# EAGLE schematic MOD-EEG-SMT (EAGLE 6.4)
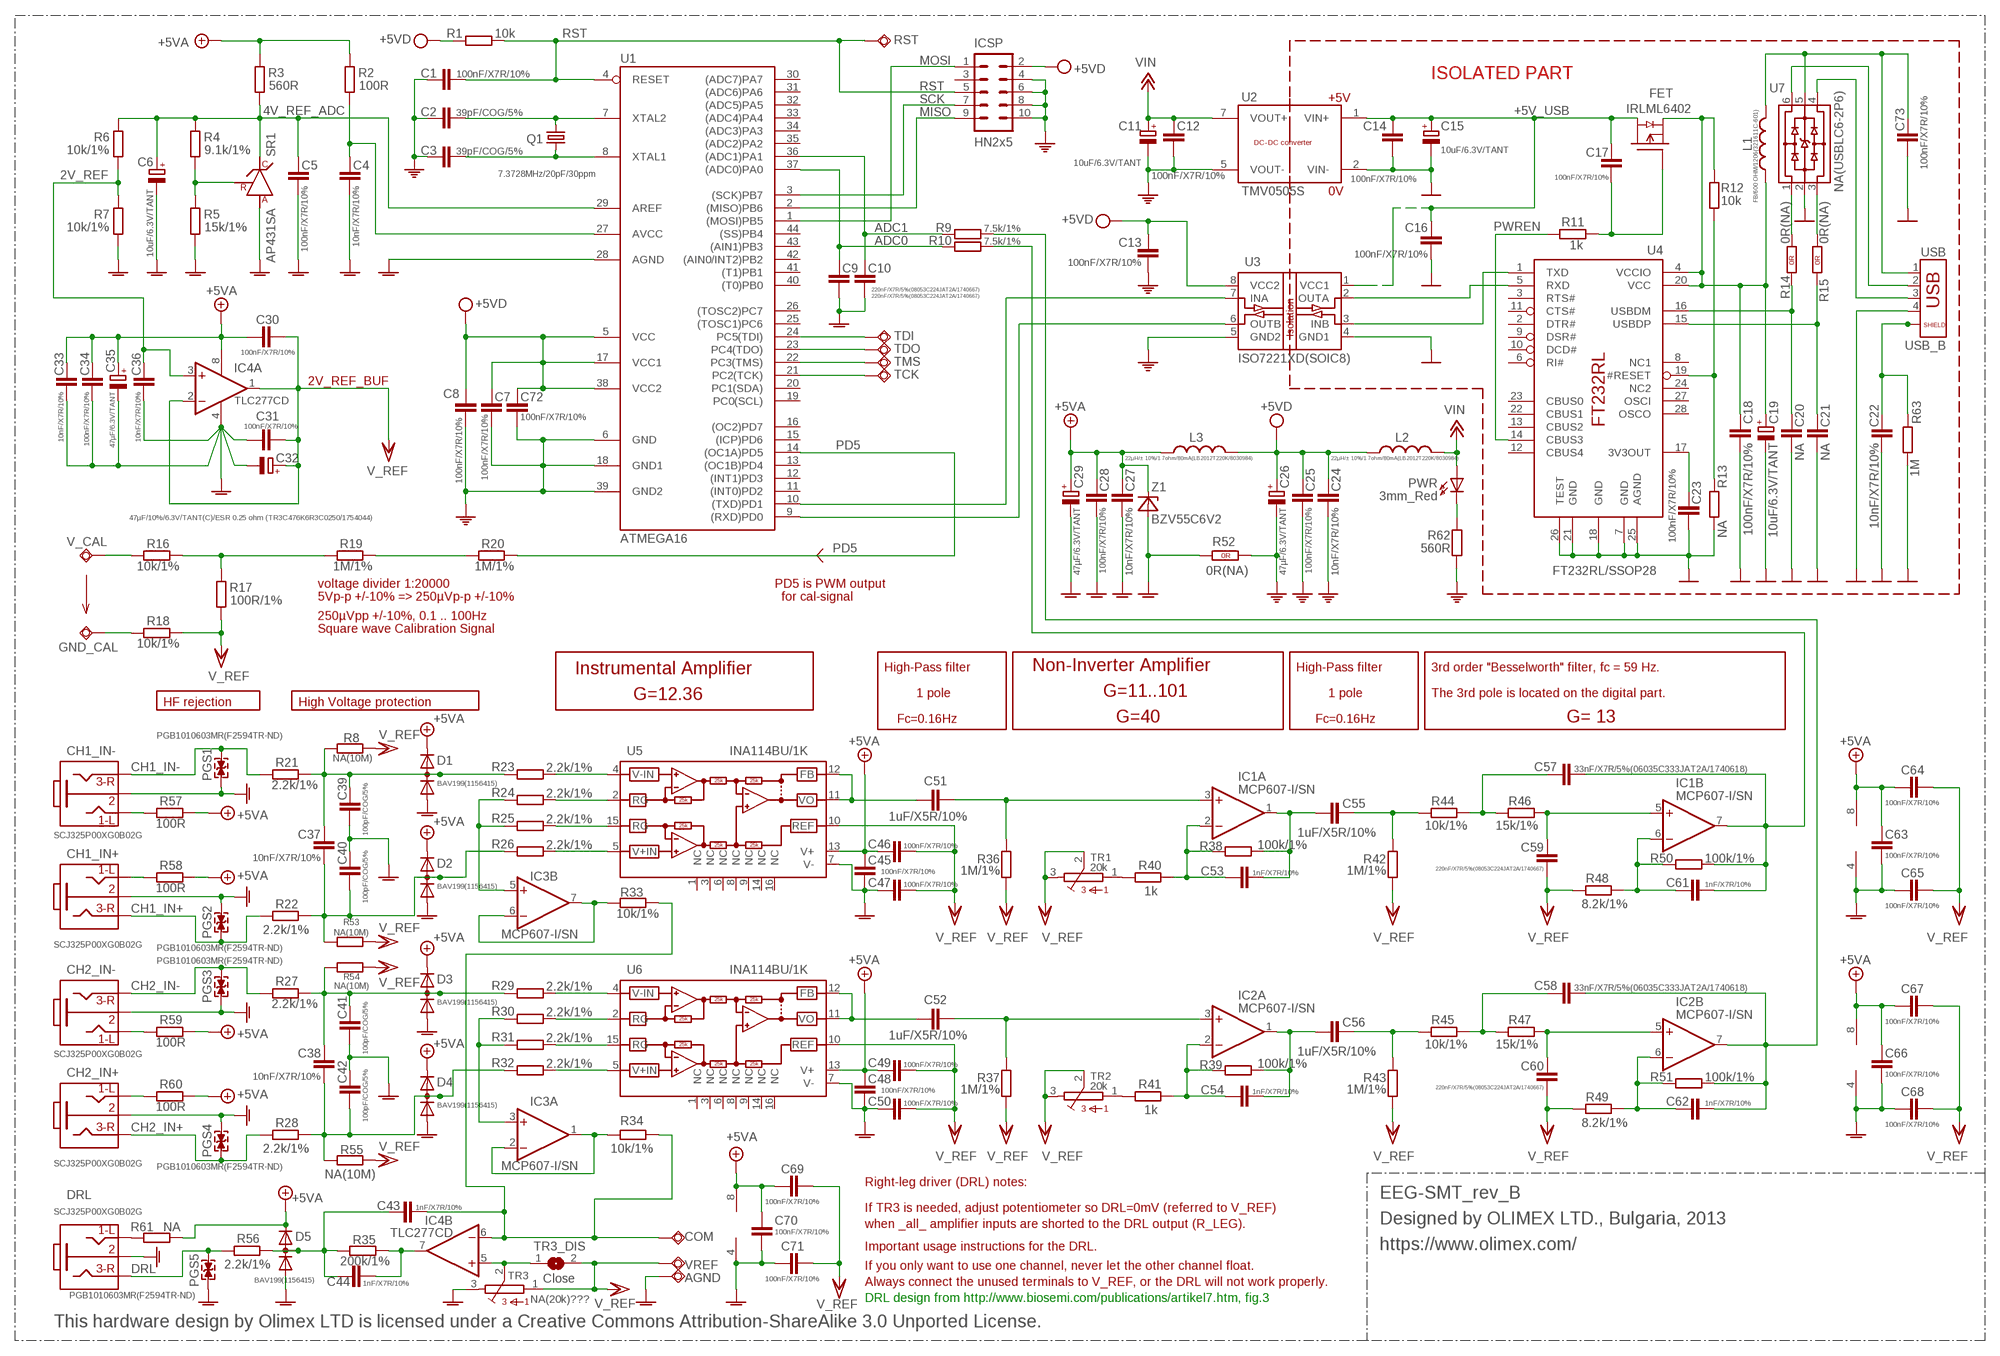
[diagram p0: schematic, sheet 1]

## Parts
AGND  TESTPAD3  [TEST_PAD40/70/SQUARE]
C1  100nF/X7R/10%  C-EUC0603_DWS  [C0603_DWS]
C2  39pF/COG/5%  C-EUC0603_DWS  [C0603_DWS]
C3  39pF/COG/5%  C-EUC0603_DWS  [C0603_DWS]
C4  10nF/X7R/10%  C-EUC0603_DWS  [C0603_DWS]
C5  100nF/X7R/10%  C-EUC0603_DWS  [C0603_DWS]
C6  10uF/6.3V/TANT  CPOL-EUCT3216  [CT3216]
C7  100nF/X7R/10%  C-EUC0603_DWS  [C0603_DWS]
C8  100nF/X7R/10%  C-EUC0603_DWS  [C0603_DWS]
C9  220nF/X7R/5%(08053C224JAT2A/1740667)  C-EUC0805_5MIL_DWS  [C0805_5MIL_DWS]
C10  220nF/X7R/5%(08053C224JAT2A/1740667)  C-EUC0805_5MIL_DWS  [C0805_5MIL_DWS]
C11  10uF/6.3V/TANT  CPOL-EUCT3216  [CT3216]
C12  100nF/X7R/10%  C-EUC0603_DWS  [C0603_DWS]
C13  100nF/X7R/10%  C-EUC0603_DWS  [C0603_DWS]
C14  100nF/X7R/10%  C-EUC0603_DWS  [C0603_DWS]
C15  10uF/6.3V/TANT  CPOL-EUCT3216  [CT3216]
C16  100nF/X7R/10%  C-EUC0603_DWS  [C0603_DWS]
C17  100nF/X7R/10%  C-EUC0603_DWS  [C0603_DWS]
C18  100nF/X7R/10%  C-EUC0603_DWS  [C0603_DWS]
C19  10uF/6.3V/TANT  CPOL-EUCT3216  [CT3216]
C20  NA  C-EUC0603_DWS_NA  [C0603_DWS_NA]
C21  NA  C-EUC0603_DWS_NA  [C0603_DWS_NA]
C22  10nF/X7R/10%  C-EUC0603_DWS  [C0603_DWS]
C23  100nF/X7R/10%  C-EUC0603_DWS  [C0603_DWS]
C24  10nF/X7R/10%  C-EUC0603_DWS  [C0603_DWS]
C25  100nF/X7R/10%  C-EUC0603_DWS  [C0603_DWS]
C26  47µF/6.3V/TANT  CPOL-EUCT3528  [CT3528]
C27  10nF/X7R/10%  C-EUC0603_DWS  [C0603_DWS]
C28  100nF/X7R/10%  C-EUC0603_DWS  [C0603_DWS]
C29  47µF/6.3V/TANT  CPOL-EUCT3528  [CT3528]
C30  100nF/X7R/10%  C-EUC0603_DWS  [C0603_DWS]
C31  100nF/X7R/10%  C-EUC0603_DWS  [C0603_DWS]
C32  47µF/10%/6.3V/TANT(C)/ESR 0.25 ohm (TR3C476K6R3C0250/1754044)  CPOL-EUCT6032  [CT6032]
C33  10nF/X7R/10%  C-EUC0603_DWS  [C0603_DWS]
C34  100nF/X7R/10%  C-EUC0603_DWS  [C0603_DWS]
C35  47µF/6.3V/TANT  CPOL-EUCT3528  [CT3528]
C36  10nF/X7R/10%  C-EUC0603_DWS  [C0603_DWS]
C37  10nF/X7R/10%  C-EUC0603_DWS  [C0603_DWS]
C38  10nF/X7R/10%  C-EUC0603_DWS  [C0603_DWS]
C39  100pF/COG/5%  C-EUC0603_DWS  [C0603_DWS]
C40  100pF/COG/5%  C-EUC0603_DWS  [C0603_DWS]
C41  100pF/COG/5%  C-EUC0603_DWS  [C0603_DWS]
C42  100pF/COG/5%  C-EUC0603_DWS  [C0603_DWS]
C43  1nF/X7R/10%  C-EUC0603_DWS  [C0603_DWS]
C44  1nF/X7R/10%  C-EUC0603_DWS  [C0603_DWS]
C45  100nF/X7R/10%  C-EUC0603_DWS  [C0603_DWS]
C46  100nF/X7R/10%  C-EUC0603_DWS  [C0603_DWS]
C47  100nF/X7R/10%  C-EUC0603_DWS  [C0603_DWS]
C48  100nF/X7R/10%  C-EUC0603_DWS  [C0603_DWS]
C49  100nF/X7R/10%  C-EUC0603_DWS  [C0603_DWS]
C50  100nF/X7R/10%  C-EUC0603_DWS  [C0603_DWS]
C51  1uF/X5R/10%  C-EUC0603_DWS  [C0603_DWS]
C52  1uF/X5R/10%  C-EUC0603_DWS  [C0603_DWS]
C53  1nF/X7R/10%  C-EUC0603_DWS  [C0603_DWS]
C54  1nF/X7R/10%  C-EUC0603_DWS  [C0603_DWS]
C55  1uF/X5R/10%  C-EUC0603_DWS  [C0603_DWS]
C56  1uF/X5R/10%  C-EUC0603_DWS  [C0603_DWS]
C57  33nF/X7R/5%(06035C333JAT2A/1740618)  C-EUC0603_DWS  [C0603_DWS]
C58  33nF/X7R/5%(06035C333JAT2A/1740618)  C-EUC0603_DWS  [C0603_DWS]
C59  220nF/X7R/5%(08053C224JAT2A/1740667)  C-EUC0805_5MIL_DWS  [C0805_5MIL_DWS]
C60  220nF/X7R/5%(08053C224JAT2A/1740667)  C-EUC0805_5MIL_DWS  [C0805_5MIL_DWS]
C61  1nF/X7R/10%  C-EUC0603_DWS  [C0603_DWS]
C62  1nF/X7R/10%  C-EUC0603_DWS  [C0603_DWS]
C63  100nF/X7R/10%  C-EUC0603_DWS  [C0603_DWS]
C64  100nF/X7R/10%  C-EUC0603_DWS  [C0603_DWS]
C65  100nF/X7R/10%  C-EUC0603_DWS  [C0603_DWS]
C66  100nF/X7R/10%  C-EUC0603_DWS  [C0603_DWS]
C67  100nF/X7R/10%  C-EUC0603_DWS  [C0603_DWS]
C68  100nF/X7R/10%  C-EUC0603_DWS  [C0603_DWS]
C69  100nF/X7R/10%  C-EUC0603_DWS  [C0603_DWS]
C70  100nF/X7R/10%  C-EUC0603_DWS  [C0603_DWS]
C71  100nF/X7R/10%  C-EUC0603_DWS  [C0603_DWS]
C72  100nF/X7R/10%  C-EUC0603_DWS  [C0603_DWS]
C73  100nF/X7R/10%  C-EUC0603_DWS  [C0603_DWS]
CH1_IN+  SCJ325P00XG0B02G  JACK-3PINPHONE_JACK-SMD  [PHONE_JACK-SMD]
CH1_IN-  SCJ325P00XG0B02G  JACK-3PINPHONE_JACK-SMD  [PHONE_JACK-SMD]
CH2_IN+  SCJ325P00XG0B02G  JACK-3PINPHONE_JACK-SMD  [PHONE_JACK-SMD]
CH2_IN-  SCJ325P00XG0B02G  JACK-3PINPHONE_JACK-SMD  [PHONE_JACK-SMD]
COM  TESTPAD3  [TEST_PAD40/70/SQUARE]
D1  BAV199(1156415)  DIODE_AC-AC_  [SOT23C(BAT54S)]
D2  BAV199(1156415)  DIODE_AC-AC_  [SOT23C(BAT54S)]
D3  BAV199(1156415)  DIODE_AC-AC_  [SOT23C(BAT54S)]
D4  BAV199(1156415)  DIODE_AC-AC_  [SOT23C(BAT54S)]
D5  BAV199(1156415)  DIODE_AC-AC_  [SOT23C(BAT54S)]
DRL  SCJ325P00XG0B02G  JACK-3PINPHONE_JACK-SMD  [PHONE_JACK-SMD]
FET  IRLML6402  [SOT23]
GND_CAL  TESTPAD3  [TEST_PAD40/70/SQUARE]
IC1  MCP607-I/SN  LM358D  [SO08]
IC2  MCP607-I/SN  LM358D  [SO08]
IC3  MCP607-I/SN  LM358D  [SO08]
IC4  TLC277CD  LM358D  [SO08]
ICSP  HN2x5  ML10ML10_NEW  [ML10_NEW]
L1  FB/600 OHM/1206(321611C-601)  L-US1206_5MIL  [L1206_5MIL]
L2  22µH/± 10%/1.7ohm/80mA(LB2012T220K/8030984)  L-USL0805_5MIL_DWS  [L0805_5MIL_DWS]
L3  22µH/± 10%/1.7ohm/80mA(LB2012T220K/8030984)  L-USL0805_5MIL_DWS  [L0805_5MIL_DWS]
PGS1  PGB1010603MR(F2594TR-ND)  [0603]
PGS2  PGB1010603MR(F2594TR-ND)  [0603]
PGS3  PGB1010603MR(F2594TR-ND)  [0603]
PGS4  PGB1010603MR(F2594TR-ND)  [0603]
PGS5  PGB1010603MR(F2594TR-ND)  [0603]
PWR  3mm_Red  LED3.0MM  [LED-3.0MM]
Q1  7.3728MHz/20pF/30ppm  HC49/S1  [HC49/SMD2_THIN]
R1  10k  R-EU_R0603_5MIL_DWS  [R0603_5MIL_DWS]
R2  100R  R-EU_R0603_5MIL_DWS  [R0603_5MIL_DWS]
R3  560R  R-EU_R0603_5MIL_DWS  [R0603_5MIL_DWS]
R4  9.1k/1%  R-EU_R0603_5MIL_DWS  [R0603_5MIL_DWS]
R5  15k/1%  R-EU_R0603_5MIL_DWS  [R0603_5MIL_DWS]
R6  10k/1%  R-EU_R0603_5MIL_DWS  [R0603_5MIL_DWS]
R7  10k/1%  R-EU_R0603_5MIL_DWS  [R0603_5MIL_DWS]
R8  NA(10M)  R-EU_R0603_5MIL_DWS  [R0603_5MIL_DWS]
R9  7.5k/1%  R-EU_R0603_5MIL_DWS  [R0603_5MIL_DWS]
R10  7.5k/1%  R-EU_R0603_5MIL_DWS  [R0603_5MIL_DWS]
R11  1k  R-EU_R0603_5MIL_DWS  [R0603_5MIL_DWS]
R12  10k  R-EU_R0603_5MIL_DWS  [R0603_5MIL_DWS]
R13  NA  R-EU_R0603_5MIL_DWS_NA  [R0603_5MIL_DWS_NA]
R14  0R(NA)  R_0R0R(NA)  [0603_0R]
R15  0R(NA)  R_0R0R(NA)  [0603_0R]
R16  10k/1%  R-EU_R0603_5MIL_DWS  [R0603_5MIL_DWS]
R17  100R/1%  R-EU_R0603_5MIL_DWS  [R0603_5MIL_DWS]
R18  10k/1%  R-EU_R0603_5MIL_DWS  [R0603_5MIL_DWS]
R19  1M/1%  R-EU_R0603_5MIL_DWS  [R0603_5MIL_DWS]
R20  1M/1%  R-EU_R0603_5MIL_DWS  [R0603_5MIL_DWS]
R21  2.2k/1%  R-EU_R0603_5MIL_DWS  [R0603_5MIL_DWS]
R22  2.2k/1%  R-EU_R0603_5MIL_DWS  [R0603_5MIL_DWS]
R23  2.2k/1%  R-EU_R0603_5MIL_DWS  [R0603_5MIL_DWS]
R24  2.2k/1%  R-EU_R0603_5MIL_DWS  [R0603_5MIL_DWS]
R25  2.2k/1%  R-EU_R0603_5MIL_DWS  [R0603_5MIL_DWS]
R26  2.2k/1%  R-EU_R0603_5MIL_DWS  [R0603_5MIL_DWS]
R27  2.2k/1%  R-EU_R0603_5MIL_DWS  [R0603_5MIL_DWS]
R28  2.2k/1%  R-EU_R0603_5MIL_DWS  [R0603_5MIL_DWS]
R29  2.2k/1%  R-EU_R0603_5MIL_DWS  [R0603_5MIL_DWS]
R30  2.2k/1%  R-EU_R0603_5MIL_DWS  [R0603_5MIL_DWS]
R31  2.2k/1%  R-EU_R0603_5MIL_DWS  [R0603_5MIL_DWS]
R32  2.2k/1%  R-EU_R0603_5MIL_DWS  [R0603_5MIL_DWS]
R33  10k/1%  R-EU_R0603_5MIL_DWS  [R0603_5MIL_DWS]
R34  10k/1%  R-EU_R0603_5MIL_DWS  [R0603_5MIL_DWS]
R35  200k/1%  R-EU_R0603_5MIL_DWS  [R0603_5MIL_DWS]
R36  1M/1%  R-EU_R0603_5MIL_DWS  [R0603_5MIL_DWS]
R37  1M/1%  R-EU_R0603_5MIL_DWS  [R0603_5MIL_DWS]
R38  100k/1%  R-EU_R0603_5MIL_DWS  [R0603_5MIL_DWS]
R39  100k/1%  R-EU_R0603_5MIL_DWS  [R0603_5MIL_DWS]
R40  1k  R-EU_R0603_5MIL_DWS  [R0603_5MIL_DWS]
R41  1k  R-EU_R0603_5MIL_DWS  [R0603_5MIL_DWS]
R42  1M/1%  R-EU_R0603_5MIL_DWS  [R0603_5MIL_DWS]
R43  1M/1%  R-EU_R0603_5MIL_DWS  [R0603_5MIL_DWS]
R44  10k/1%  R-EU_R0603_5MIL_DWS  [R0603_5MIL_DWS]
R45  10k/1%  R-EU_R0603_5MIL_DWS  [R0603_5MIL_DWS]
R46  15k/1%  R-EU_R0603_5MIL_DWS  [R0603_5MIL_DWS]
R47  15k/1%  R-EU_R0603_5MIL_DWS  [R0603_5MIL_DWS]
R48  8.2k/1%  R-EU_R0603_5MIL_DWS  [R0603_5MIL_DWS]
R49  8.2k/1%  R-EU_R0603_5MIL_DWS  [R0603_5MIL_DWS]
R50  100k/1%  R-EU_R0603_5MIL_DWS  [R0603_5MIL_DWS]
R51  100k/1%  R-EU_R0603_5MIL_DWS  [R0603_5MIL_DWS]
R52  0R(NA)  R_0R0R(NA)  [0603_0R]
R53  NA(10M)  R-EU_R0603_5MIL_DWS  [R0603_5MIL_DWS]
R54  NA(10M)  R-EU_R0603_5MIL_DWS  [R0603_5MIL_DWS]
R55  NA(10M)  R-EU_R0603_5MIL_DWS  [R0603_5MIL_DWS]
R56  2.2k/1%  R-EU_R0603_5MIL_DWS  [R0603_5MIL_DWS]
R57  100R  R-EU_R0603_5MIL_DWS  [R0603_5MIL_DWS]
R58  100R  R-EU_R0603_5MIL_DWS  [R0603_5MIL_DWS]
R59  100R  R-EU_R0603_5MIL_DWS  [R0603_5MIL_DWS]
R60  100R  R-EU_R0603_5MIL_DWS  [R0603_5MIL_DWS]
R61  NA  R-EU_R0603_5MIL_DWS_NA  [R0603_5MIL_DWS_NA]
R62  560R  R-EU_R0603_5MIL_DWS  [R0603_5MIL_DWS]
R63  1M  R-EU_R0603_5MIL_DWS  [R0603_5MIL_DWS]
RST  TESTPAD80/30  [SMD80/30]
SR1  AP431SA  TL431'''  [SOT-23]
TCK  TESTPAD80/30  [SMD80/30]
TDI  TESTPAD80/30  [SMD80/30]
TDO  TESTPAD80/30  [SMD80/30]
TMS  TESTPAD80/30  [SMD80/30]
TR1  20k  S64Y  [S64Y]
TR2  20k  S64Y  [S64Y]
TR3  NA(20k)???  S64Y  [S64Y]
TR3_DIS  Close  SJSJ_SMALLER  [SJ_1_SMALLER]
U1  ATMEGA16  [44TQFP]
U2  TMV0505S  TMV0505  [TMADCDC]
U3  ISO7221XD(SOIC8)  ISO7221XD  [SO-8_ISOLATE]
U4  FT232RL/SSOP28  FT232RLSSOP28  [SSOP28]
U5  INA114BU/1K  [SO16]
U6  INA114BU/1K  [SO16]
U7  NA(USBLC6-2P6)  USBLC6-2  [USBLC6-2P6]
USB  USB_B  USB_SHIELD  [USB_NEAR_BLACK]
V_CAL  TESTPAD3  [TEST_PAD40/70/SQUARE]
VREF  TESTPAD3  [TEST_PAD40/70/SQUARE]
Z1  BZV55C6V2  ZDIOD-SMD  [MINI-MELF]

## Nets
2V_REF: C36.1 IC4.3(A:+IN) R6.1 R7.2
4V_REF_ADC: C5.1 C6.+ R3.1 R4.2 R6.2 SR1.1(C) U1.29(AREF)
+5V: C27.1 C28.1 C29.+ C30.2 C33.1 C34.1 C35.+ C45.1 C46.1 C48.1 C49.1 C63.1 C64.1 C66.1 C67.1 C69.1 C70.1 D1.2(K) D2.2(K) D3.2(K) D4.2(K) D5.2(K) IC1.8(P:V+) IC2.8(P:V+) IC3.8(P:V+) IC4.8(P:V+) L3.2 R2.2 R3.2 R57.2 R58.2 R59.2 R60.2 R61.2 U5.13(V+) U6.13(V+) Z1.1(C) ; supply symbol labelled +5VA
+5V_USB: C14.1 C15.+ C16.1 C17.1 FET.3(D) U2.1(VIN+) U3.1(VCC1)
+12V: C11.+ C12.1 L2.1 PWR.A U2.7(VOUT+) ; supply symbol labelled VIN
ADC0: C9.1 R10.1 U1.37((ADC0)PA0)
ADC1: C10.1 R9.1 U1.36((ADC1)PA1)
CH1_IN+: CH1_IN+.2 PGS2.1 R22.1
CH1_IN-: CH1_IN-.2 PGS1.2 R21.1
CH2_IN+: CH2_IN+.2 PGS4.1 R28.1
CH2_IN-: CH2_IN-.2 PGS3.2 R27.1
DRL: DRL.2 PGS5.2 R56.1
GND: C14.2 C15.- C16.2 C18.2 C19.- C20.2 C21.2 C22.2 C23.2 C73.2 R13.1 R63.1 U2.2(VIN-) U3.4(GND1) U4.7(GND) U4.18(GND) U4.21(GND) U4.25(AGND) U4.26(TEST) U7.2 USB.4
GNDA [pwr]: AGND.P$1(PP) C4.2 C5.2 C6.- C9.2 C10.2 C27.2 C28.2 C29.- C31.2 C32.- C33.2 C34.2 C35.- C36.2 C39.1 C40.2 C41.1 C42.2 C45.2 C47.1 C48.2 C50.1 C63.2 C65.1 C66.2 C68.1 C70.2 C71.1 CH1_IN+.1 CH1_IN-.1 CH2_IN+.1 CH2_IN-.1 D1.1(A) D2.1(A) D3.1(A) D4.1(A) D5.1(A) DRL.1 IC1.4(P:V-) IC2.4(P:V-) IC3.4(P:V-) IC4.4(P:V-) PGS1.1 PGS2.2 PGS3.1 PGS4.2 PGS5.1 R5.1 R7.1 R52.1(1.1) SR1.3(A) TR3.3 U1.28(AGND) U5.7(V-) U6.7(V-) Z1.2(A)
MISO: ICSP.9 U1.2((MISO)PB6)
MOSI: ICSP.1 U1.1((MOSI)PB5)
N$1: R14.1(1.1) U7.1
N$2: R15.1(1.1) U7.3
N$3: TDI.P$1(PP) U1.24(PC5(TDI))
N$4: TDO.P$1(PP) U1.23(PC4(TDO))
N$5: TMS.P$1(PP) U1.22(PC3(TMS))
N$6: TCK.P$1(PP) U1.21(PC2(TCK))
N$7: CH1_IN-.5 R57.1
N$8: CH1_IN+.5 R58.1
N$9: C43.2 C44.2 D5.3(AK) R35.1 R56.2
N$10: CH2_IN+.5 R60.1
N$11: CH2_IN-.5 R59.1
N$12: DRL.5 R61.1
N$15: PWR.K(C) R62.2
N$16: U3.2(OUTA) U4.5(RXD)
N$17: C22.1 R63.2 USB.P$1 USB.P$2
N$18: U7.6 USB.2
N$20: U3.3(INB) U4.1(TXD)
N$21: C4.1 R2.1 U1.27(AVCC)
N$22: R4.1 R5.2 SR1.2(R)
N$23: U1.10((TXD)PD1) U3.7(INA)
N$24: U1.9((RXD)PD0) U3.6(OUTB)
N$25: U7.4 USB.3
N$26: C73.1 L1.1 U7.5 USB.1
N$27: C3.1 Q1.2 U1.8(XTAL1)
N$28: C2.1 Q1.1 U1.7(XTAL2)
N$29: R40.2 TR1.1
N$30: R41.2 TR2.1
N$35: R12.1 R13.2 U4.19(#RESET)
N$78: C23.1 U4.17(3V3OUT)
N$79: C18.1 C19.+ FET.2(S) L1.2 R12.2 U4.4(VCCIO) U4.20(VCC)
N$81: C55.2 R42.1 R44.1
N$83: C51.1 U5.11(VO) U5.12(FB)
N$84: R23.1 U5.4(V-IN)
N$88: R24.1 U5.2(RG)
N$92: C37.1 C40.1 D2.3(AK) R22.2 R26.2 R53.2
N$93: C37.2 C39.2 D1.3(AK) R8.2 R21.2 R23.2
N$94: C38.1 C42.1 D4.3(AK) R28.2 R32.2 R55.2
N$95: C38.2 C41.2 D3.3(AK) R27.2 R29.2 R54.2
N$101: R25.1 U5.15(RG)
N$102: C51.2 IC1.3(A:+IN) R36.1
N$103: IC3.5(B:+IN) R24.2 R25.2
N$104: C53.2 C55.1 IC1.1(A:OUT) R38.2
N$105: C53.1 IC1.2(A:-IN) R38.1 R40.1
N$106: R26.1 U5.5(V+IN)
N$107: C59.1 IC1.5(B:+IN) R46.2
N$108: C57.1 R44.2 R46.1
N$109: C57.2 C61.2 IC1.7(B:OUT) R10.2 R50.2
N$110: C61.1 IC1.6(B:-IN) R48.1 R50.1
N$113: C52.2 IC2.3(A:+IN) R37.1
N$125: C54.2 C56.1 IC2.1(A:OUT) R39.2
N$126: C54.1 IC2.2(A:-IN) R39.1 R41.1
N$127: C60.1 IC2.5(B:+IN) R47.2
N$128: C58.1 R45.2 R47.1
N$129: C58.2 C62.2 IC2.7(B:OUT) R9.2 R51.2
N$130: C62.1 IC2.6(B:-IN) R49.1 R51.1
N$131: C56.2 R43.1 R45.1
N$133: C52.1 U6.11(VO) U6.12(FB)
N$134: R30.1 U6.2(RG)
N$135: R31.1 U6.15(RG)
N$136: IC3.3(A:+IN) R30.2 R31.2
N$137: R29.1 U6.4(V-IN)
N$138: R32.1 U6.5(V+IN)
N$139: IC3.1(A:OUT) IC3.2(A:-IN) R34.2
N$140: IC3.6(B:-IN) IC3.7(B:OUT) R33.2
N$141: IC4.5(B:+IN) TR3.2 TR3_DIS.1
N$142: C44.1 IC4.7(B:OUT) R35.2
N$144: R19.2 R20.1
N$145: C43.1 COM.P$1(PP) IC4.6(B:-IN) R33.1 R34.1
N$146: R16.2 R17.2 R19.1
N$148: R16.1 V_CAL.P$1(PP)
N$149: GND_CAL.P$1(PP) R18.1
N$168: C17.2 FET.1(G) R11.2
PD5: R20.2 U1.14((OC1A)PD5)
PE: C1.2 C2.2 C3.2 C7.2 C8.2 C11.- C12.2 C13.2 C24.2 C25.2 C26.- C72.2 ICSP.4 ICSP.6 ICSP.8 ICSP.10 R52.2(1.2) R62.1 U1.6(GND) U1.18(GND1) U1.39(GND2) U2.5(VOUT-) U3.5(GND2)
PWREN: R11.1 U4.14(CBUS3)
RST: C1.1 ICSP.5 R1.2 RST.P$1(PP) U1.4(RESET)
SCK: ICSP.7 U1.3((SCK)PB7)
USBDM: C20.1 R14.2(1.2) U4.16(USBDM)
USBDP: C21.1 R15.2(1.2) U4.15(USBDP)
VCC/2: C30.1 C31.1 C32.+ C46.2 C47.2 C49.2 C50.2 C59.2 C60.2 C64.2 C65.2 C67.2 C68.2 C69.2 C71.2 IC4.1(A:OUT) IC4.2(A:-IN) R8.1 R17.1 R18.2 R36.2 R37.2 R42.2 R43.2 R48.2 R49.2 R53.1 R54.1 R55.1 TR1.2 TR1.3 TR2.2 TR2.3 TR3.1 TR3_DIS.2 U5.10(REF) U6.10(REF) VREF.P$1(PP) ; supply symbol labelled V_REF
VPP: C7.1 C8.1 C13.1 C24.1 C25.1 C26.+ C72.1 ICSP.2 L2.2 L3.1 R1.1 U1.5(VCC) U1.17(VCC1) U1.38(VCC2) U3.8(VCC2) ; supply symbol labelled +5VD
Unconnected: ICSP.3 U1.11((INT0)PD2) U1.12((INT1)PD3) U1.13((OC1B)PD4) U1.15((ICP)PD6) U1.16((OC2)PD7) U1.19(PC0(SCL)) U1.20(PC1(SDA)) U1.25((TOSC1)PC6) U1.26((TOSC2)PC7) U1.30((ADC7)PA7) U1.31((ADC6)PA6) U1.32((ADC5)PA5) U1.33((ADC4)PA4) U1.34((ADC3)PA3) U1.35((ADC2)PA2) U1.40((T0)PB0) U1.41((T1)PB1) U1.42((AIN0/INT2)PB2) U1.43((AIN1)PB3) U1.44((SS)PB4) U4.2(DTR#) U4.3(RTS#) U4.6(RI#) U4.8(NC1) U4.9(DSR#) U4.10(DCD#) U4.11(CTS#) U4.12(CBUS4) U4.13(CBUS2) U4.22(CBUS1) U4.23(CBUS0) U4.24(NC2) U4.27(OSCI) U4.28(OSCO) U5.1(NC) U5.3(NC) U5.6(NC) U5.8(NC) U5.9(NC) U5.14(NC) U5.16(NC) U6.1(NC) U6.3(NC) U6.6(NC) U6.8(NC) U6.9(NC) U6.14(NC) U6.16(NC)

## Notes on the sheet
- ISOLATED PART
- +5V
- 0V
- 2V_REF_BUF
- voltage divider 1:20000 | PD5 is PWM output
- 5Vp-p +/-10% => 250µVp-p +/-10% | for cal-signal
- 250µVpp +/-10%, 0.1 .. 100Hz
- Square wave Calibration Signal
- Instrumental Amplifier | High-Pass filter | Non-Inverter Amplifier | High-Pass filter | 3rd order "Besselworth" filter, fc = 59 Hz.
- HF rejection | High Voltage protection | G=12.36 | 1 pole | G=11..101 | 1 pole | The 3rd pole is located on the digital part.
- Fc=0.16Hz | G=40 | Fc=0.16Hz | G= 13
- Right-leg driver (DRL) notes:
- EEG-SMT_rev_B
- If TR3 is needed, adjust potentiometer so DRL=0mV (referred to V_REF)
- when _all_ amplifier inputs are shorted to the DRL output (R_LEG). | Designed by OLIMEX LTD., Bulgaria, 2013
- Important usage instructions for the DRL. | https://www.olimex.com/
- If you only want to use one channel, never let the other channel float.
- Always connect the unused terminals to V_REF, or the DRL will not work properly.
- DRL design from http://www.biosemi.com/publications/artikel7.htm, fig.3
- This hardware design by Olimex LTD is licensed under a Creative Commons Attribution-ShareAlike 3.0 Unported License.

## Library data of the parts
AGND COM GND_CAL RST TCK TDI TDO TMS V_CAL VREF = gogo:TESTPAD: drill 40mils, diameter 70mils
C1-C5 C7-C10 C12-C14 C16-C18 C20-C25 C27 C28 C30 C31 C33 C34 C36-C73 = rcl:C-EU: CAPACITOR, European symbol
C6 C11 C15 C19 C26 C29 C32 C35 = rcl:CPOL-EU: POLARIZED CAPACITOR, European symbol
CH1_IN+ CH1_IN- CH2_IN+ CH2_IN- DRL = gogo:JACK-3PIN
D1-D5 = semicon-smd-ipc:DIODE_AC-AC_: DUAL DIODE
FET = gogo:IRLML6402
IC1-IC4 = linear:LM358: OP AMP
ICSP = con-harting-ml:ML10: HARTING
L1-L3 = rcl:L-US: INDUCTOR, American symbol
PGS1-PGS5 = OLIMEX_DISCRET:PGB1010603MR: PulseGuard® Suppressors
PWR = DOUBLE-SIDE:LED
Q1 = crystal:HC49/S: CRYSTAL
R1-R13 R16-R51 R53-R63 = rcl:R-EU_: RESISTOR, European symbol
R14 R15 R52 = OLIMEX_DISCRET:R_0R
SR1 = OLIMEX_IC:TL431: TL431 Programmable Shunt Regulator Features: -> Programmable Output Voltage to 36 Volts -> Low Dynamic Output Impedance 0.20 Typical -> Sink Current Capability of 1.0 to 100mA -> Equivalent Full-Range Temperature Coefficient of 50ppm/°C Typical -> Temperature Compensated For Operation Over Full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
TR1-TR3 = TRIMPOT:S64Y
TR3_DIS = jumper:SJ: SMD solder JUMPER
U1 = gogo:ATMEGA16
U2 = MODEEG:TMV0505
U3 = OLIMEX_IC:ISO7221XD: ISO7221 - dual-channel digital isolator FEATURES: -> 1, 25, and 150-Mbps Signaling Rate Options; -> Low Channel-to-Channel Output Skew - 1 ns max; -> Low Pulse-Width Distortion (PWD) - 1 ns max; -> Low Jitter Content - 1 ns Typ at 150 Mbps; -> Typical 25-Year Life at Rated Voltage; -> 4000-Vpeak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
U4 = OLIMEX_IC:FT232RL
U5 U6 = OLIMEX_IC:INA114
U7 = OLIMEX_IC:USBLC6-2
USB = OLIMEX_CONNECTORS:USB_SHIELD
Z1 = gogo:ZDIOD-SMD

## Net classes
1 pwr: width 0.4 mm, clearance 0.23 mm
